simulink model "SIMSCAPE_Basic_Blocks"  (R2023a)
settings: Solver=VariableStepAuto  StartTime=0.0  StopTime=10.0  RelTol=1e-3
model workspace (MAT data in the model file):
  xx = 'A'
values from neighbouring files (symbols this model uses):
  R = 1    [Electrical_Transformer_EQN.m]    (also in Electrical_Transformer_SLX_m.m; Mechanical_Transmission_EQN.m; Mechanical_Transmission_SLX_m.m; Mechanical_system_EQN.m)
undefined symbols (not defined in the file or in its folder): Ap, eTr, mGi
libraries: fl_lib x28, nesl_utility x4

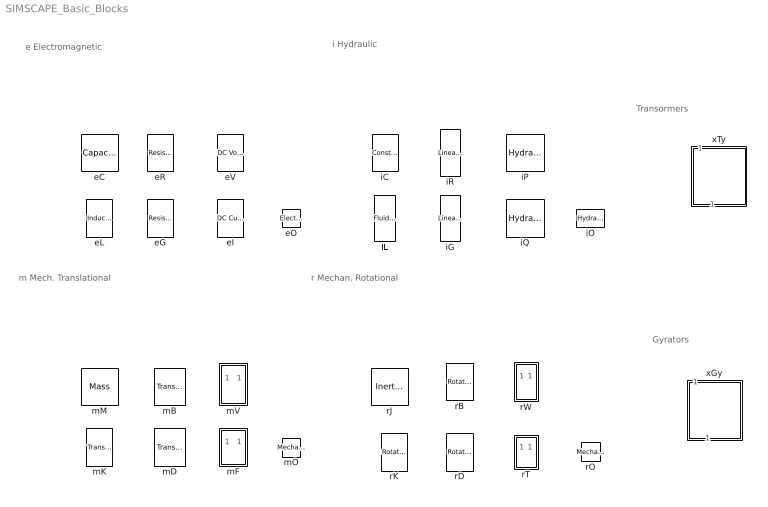
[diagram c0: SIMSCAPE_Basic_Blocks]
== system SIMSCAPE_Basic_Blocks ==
  note: m Mech. Translational
  note: r Mechan. Rotational
  note: i Hydraulic
  note: e Electromagnetic
  note: Transormers
  note: Gyrators
  eC : fl_lib/Electrical/Electrical Elements/Capacitor  c=1e-6 F  r=1e-6 Ohm  g=0 1/Ohm  i_specify=off  i_priority=None  i=0 A  i_nominal_specify=off  i_nominal_unit=A  i_nominal_value=1  v_specify=off  v_priority=None  v=0 V  v_nominal_specify=off  v_nominal_unit=V  v_nominal_value=1  vc_specify=off  vc_priority=High  vc=0 V  vc_nominal_specify=off  vc_nominal_unit=V  vc_nominal_value=1
  eG : fl_lib/Electrical/Electrical Elements/Resistor  R=1 Ohm  i_specify=off  i_priority=None  i=0 A  i_nominal_specify=off  i_nominal_unit=A  i_nominal_value=1  v_specify=off  v_priority=None  v=0 V  v_nominal_specify=off  v_nominal_unit=V  v_nominal_value=1
  eI : fl_lib/Electrical/Electrical Sources/DC Current Source  i0=1 A
  eL : fl_lib/Electrical/Electrical Elements/Inductor  l=1e-6 H  r=0 Ohm  g=1e-9 1/Ohm  i_specify=off  i_priority=None  i=0 A  i_nominal_specify=off  i_nominal_unit=A  i_nominal_value=1  v_specify=off  v_priority=None  v=0 V  v_nominal_specify=off  v_nominal_unit=V  v_nominal_value=1  i_L_specify=off  i_L_priority=High  i_L=0 A  i_L_nominal_specify=off  i_L_nominal_unit=A  i_L_nominal_value=1
  eO : fl_lib/Electrical/Electrical Elements/Electrical Reference
  eR : fl_lib/Electrical/Electrical Elements/Resistor  R=1 Ohm  i_specify=off  i_priority=None  i=0 A  i_nominal_specify=off  i_nominal_unit=A  i_nominal_value=1  v_specify=off  v_priority=None  v=0 V  v_nominal_specify=off  v_nominal_unit=V  v_nominal_value=1
  eV : fl_lib/Electrical/Electrical Sources/DC Voltage Source  v0=1 V
  iC : fl_lib/Hydraulic/Hydraulic Elements/Constant Volume Hydraulic Chamber  ch_sp=foundation.enum.chamberGeometry.volume  wall_type=foundation.enum.chamber_spec.rigid  ch_volume=1e-4 m^3  d_in=1e-2 m  length=1 m  pr_r_coef=1.2e-12 m/Pa  time_const=0.01 s  k_sh=1.4  pressure_specify=off  pressure_priority=High  pressure=0 Pa  pressure_nominal_specify=off  pressure_nominal_unit=Pa  pressure_nominal_value=1  diameter_incr_specify=off  diameter_incr_priority=High  diameter_incr=0 m  diameter_incr_nominal_specify=off  diameter_incr_nominal_unit=m  diameter_incr_nominal_value=1  flow_rate_specify=off  flow_rate_priority=None  flow_rate=1e-3 m^3/s  flow_rate_nominal_specify=off  flow_rate_nominal_unit=m^3/s  flow_rate_nominal_value=1
  iG : fl_lib/Hydraulic/Hydraulic Elements/Linear Hydraulic Resistance  resistance=10e9 Pa*s/m^3  q_specify=off  q_priority=None  q=1e-3 m^3/s  q_nominal_specify=off  q_nominal_unit=m^3/s  q_nominal_value=1  p_specify=off  p_priority=None  p=0 Pa  p_nominal_specify=off  p_nominal_unit=Pa  p_nominal_value=1
  iL : fl_lib/Hydraulic/Hydraulic Elements/Fluid Inertia  area=0.8e-4 m^2  length=1 m  q_specify=off  q_priority=High  q=1e-3 m^3/s  q_nominal_specify=off  q_nominal_unit=m^3/s  q_nominal_value=1  p_specify=off  p_priority=None  p=0 Pa  p_nominal_specify=off  p_nominal_unit=Pa  p_nominal_value=1
  iO : fl_lib/Hydraulic/Hydraulic Elements/Hydraulic Reference
  iP : fl_lib/Hydraulic/Hydraulic Sources/Hydraulic Constant Pressure Source  commanded_pressure=10e5 Pa
  iQ : fl_lib/Hydraulic/Hydraulic Sources/Hydraulic Constant Flow Rate Source  commanded_flow_rate=0.001 m^3/s
  iR : fl_lib/Hydraulic/Hydraulic Elements/Linear Hydraulic Resistance  resistance=10e9 Pa*s/m^3  q_specify=off  q_priority=None  q=1e-3 m^3/s  q_nominal_specify=off  q_nominal_unit=m^3/s  q_nominal_value=1  p_specify=off  p_priority=None  p=0 Pa  p_nominal_specify=off  p_nominal_unit=Pa  p_nominal_value=1
  mB : fl_lib/Mechanical/Translational Elements/Translational Damper  D=100 N*s/m  v_specify=off  v_priority=None  v=0 m/s  v_nominal_specify=off  v_nominal_unit=m/s  v_nominal_value=1  f_specify=off  f_priority=None  f=0 N  f_nominal_specify=off  f_nominal_unit=N  f_nominal_value=1
  mD : fl_lib/Mechanical/Translational Elements/Translational Damper  D=100 N*s/m  v_specify=off  v_priority=None  v=0 m/s  v_nominal_specify=off  v_nominal_unit=m/s  v_nominal_value=1  f_specify=off  f_priority=None  f=0 N  f_nominal_specify=off  f_nominal_unit=N  f_nominal_value=1
  mF : Subsystem  mask{mF='Fa'}
      mask prompts: mF "Output variable"
  mK : fl_lib/Mechanical/Translational Elements/Translational Spring  spr_rate=1000 N/m  v_specify=off  v_priority=None  v=0 m/s  v_nominal_specify=off  v_nominal_unit=m/s  v_nominal_value=1  f_specify=off  f_priority=None  f=0 N  f_nominal_specify=off  f_nominal_unit=N  f_nominal_value=1  x_specify=off  x_priority=High  x=0 m  x_nominal_specify=off  x_nominal_unit=m  x_nominal_value=1
  mM : fl_lib/Mechanical/Translational Elements/Mass  mass=1 kg  num_ports=foundation.enum.numPorts2.one  v_specify=off  v_priority=High  v=0 m/s  v_nominal_specify=off  v_nominal_unit=m/s  v_nominal_value=1  f_specify=off  f_priority=None  f=0 N  f_nominal_specify=off  f_nominal_unit=N  f_nominal_value=1
  mO : fl_lib/Mechanical/Translational Elements/Mechanical Translational Reference
  mV : Subsystem  mask{mV='Va'}
      mask prompts: mV "Output variable"
  rB : fl_lib/Mechanical/Rotational Elements/Rotational Damper  D=0.001 N*m*s/rad  w_specify=off  w_priority=None  w=0 rad/s  w_nominal_specify=off  w_nominal_unit=rad/s  w_nominal_value=1  t_specify=off  t_priority=None  t=0 N*m  t_nominal_specify=off  t_nominal_unit=N*m  t_nominal_value=1
  rD : fl_lib/Mechanical/Rotational Elements/Rotational Damper  D=0.001 N*m*s/rad  w_specify=off  w_priority=None  w=0 rad/s  w_nominal_specify=off  w_nominal_unit=rad/s  w_nominal_value=1  t_specify=off  t_priority=None  t=0 N*m  t_nominal_specify=off  t_nominal_unit=N*m  t_nominal_value=1
  rJ : fl_lib/Mechanical/Rotational Elements/Inertia  inertia=0.01 kg*m^2  num_ports=foundation.enum.numPorts2.one  w_specify=off  w_priority=High  w=0 rad/s  w_nominal_specify=off  w_nominal_unit=rad/s  w_nominal_value=1  t_specify=off  t_priority=None  t=0 N*m  t_nominal_specify=off  t_nominal_unit=N*m  t_nominal_value=1
  rK : fl_lib/Mechanical/Rotational Elements/Rotational Spring  spr_rate=10 N*m/rad  w_specify=off  w_priority=None  w=0 rad/s  w_nominal_specify=off  w_nominal_unit=rad/s  w_nominal_value=1  t_specify=off  t_priority=None  t=0 N*m  t_nominal_specify=off  t_nominal_unit=N*m  t_nominal_value=1  phi_specify=off  phi_priority=High  phi=0 rad  phi_nominal_specify=off  phi_nominal_unit=rad  phi_nominal_value=1
  rO : fl_lib/Mechanical/Rotational Elements/Mechanical Rotational Reference
  rT : Subsystem  mask{rT='Ta'}
      mask prompts: rT "Output variable"
  rW : Subsystem  mask{rW='Wa'}
      mask prompts: rW "Output variable"
  xGy : Subsystem  mask{Gyrator_type=mGi, G_type=F2=K*E1, xGy=Ap}
      mask prompts: Gyrator_type "Type of Gytator"; G_type "Type of relation"; xGy "Name of parameter K"
  xTy : Subsystem  mask{Transformer_type=eTr, T_type=E2=K*E1, xTy=R}
      mask prompts: Transformer_type "Type of Transformer"; T_type "Type of relation"; xTy "Name of parameter K"

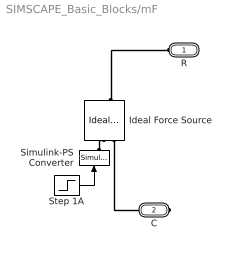
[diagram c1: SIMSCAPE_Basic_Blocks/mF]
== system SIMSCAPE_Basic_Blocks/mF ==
  Ideal Force Source : fl_lib/Mechanical/Mechanical Sources/Ideal Force Source
  Simulink-PS Converter : nesl_utility/Simulink-PS Converter  PhysicalDomain=network_engine_domain  SubClassName=ps_input  LeftPortType=input  RightPortType=output  PseudoPeriodic=off  Frequencies=[]  NoiseDistribution=none  NoiseParameters=[]  Unit=1  AffineConversion=off  FilteringAndDerivatives=zero  SimscapeFilterOrder=1  InputFilterTimeConstant=.001  UdotUserProvided=0
  Step 1A : Step  After=100  SampleTime=0
  R : PMIOPort  Side=Left
  C : PMIOPort  Port=2  Side=Right
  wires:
  Step 1A/1 -> Simulink-PS Converter/1
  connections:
  Ideal Force Source/RConn2 -- C/RConn1
  Ideal Force Source/LConn1 -- R/RConn1
  Simulink-PS Converter/RConn1 -- Ideal Force Source/RConn1

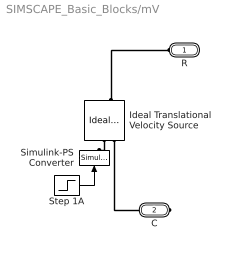
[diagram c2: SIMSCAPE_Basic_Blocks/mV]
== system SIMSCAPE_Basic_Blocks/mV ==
  Ideal Translational Velocity Source : fl_lib/Mechanical/Mechanical Sources/Ideal Translational Velocity Source
  Simulink-PS Converter : nesl_utility/Simulink-PS Converter  PhysicalDomain=network_engine_domain  SubClassName=ps_input  LeftPortType=input  RightPortType=output  PseudoPeriodic=off  Frequencies=[]  NoiseDistribution=none  NoiseParameters=[]  Unit=1  AffineConversion=off  FilteringAndDerivatives=zero  SimscapeFilterOrder=1  InputFilterTimeConstant=.001  UdotUserProvided=0
  Step 1A : Step  After=100  SampleTime=0
  R : PMIOPort  Side=Left
  C : PMIOPort  Port=2  Side=Right
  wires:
  Step 1A/1 -> Simulink-PS Converter/1
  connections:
  Ideal Translational Velocity Source/RConn2 -- C/RConn1
  Ideal Translational Velocity Source/LConn1 -- R/RConn1
  Ideal Translational Velocity Source/RConn1 -- Simulink-PS Converter/RConn1

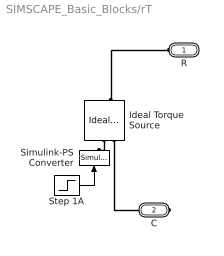
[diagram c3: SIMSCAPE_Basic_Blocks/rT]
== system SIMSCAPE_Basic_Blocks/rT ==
  Ideal Torque Source : fl_lib/Mechanical/Mechanical Sources/Ideal Torque Source
  Simulink-PS Converter : nesl_utility/Simulink-PS Converter  PhysicalDomain=network_engine_domain  SubClassName=ps_input  LeftPortType=input  RightPortType=output  PseudoPeriodic=off  Frequencies=[]  NoiseDistribution=none  NoiseParameters=[]  Unit=1  AffineConversion=off  FilteringAndDerivatives=zero  SimscapeFilterOrder=1  InputFilterTimeConstant=.001  UdotUserProvided=0
  Step 1A : Step  After=100  SampleTime=0
  R : PMIOPort  Side=Left
  C : PMIOPort  Port=2  Side=Right
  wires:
  Step 1A/1 -> Simulink-PS Converter/1
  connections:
  Ideal Torque Source/RConn1 -- Simulink-PS Converter/RConn1
  Ideal Torque Source/LConn1 -- R/RConn1
  Ideal Torque Source/RConn2 -- C/RConn1

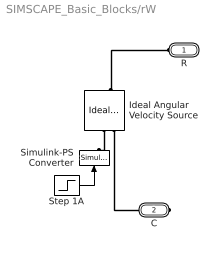
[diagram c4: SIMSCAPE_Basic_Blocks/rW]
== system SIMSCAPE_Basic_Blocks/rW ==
  Ideal Angular Velocity Source : fl_lib/Mechanical/Mechanical Sources/Ideal Angular Velocity Source
  Simulink-PS Converter : nesl_utility/Simulink-PS Converter  PhysicalDomain=network_engine_domain  SubClassName=ps_input  LeftPortType=input  RightPortType=output  PseudoPeriodic=off  Frequencies=[]  NoiseDistribution=none  NoiseParameters=[]  Unit=1  AffineConversion=off  FilteringAndDerivatives=zero  SimscapeFilterOrder=1  InputFilterTimeConstant=.001  UdotUserProvided=0
  Step 1A : Step  After=100  SampleTime=0
  R : PMIOPort  Side=Left
  C : PMIOPort  Port=2  Side=Right
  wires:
  Step 1A/1 -> Simulink-PS Converter/1
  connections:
  Ideal Angular Velocity Source/RConn2 -- C/RConn1
  Ideal Angular Velocity Source/LConn1 -- R/RConn1
  Ideal Angular Velocity Source/RConn1 -- Simulink-PS Converter/RConn1

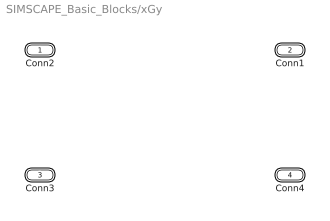
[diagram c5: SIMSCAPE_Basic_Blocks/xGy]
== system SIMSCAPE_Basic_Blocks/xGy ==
  Conn2 : PMIOPort  Side=Left
  Conn1 : PMIOPort  Port=2  Side=Left
  Conn3 : PMIOPort  Port=3  Side=Right
  Conn4 : PMIOPort  Port=4  Side=Right

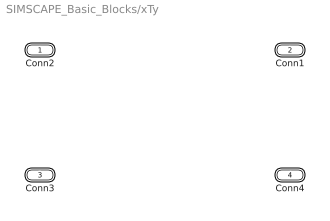
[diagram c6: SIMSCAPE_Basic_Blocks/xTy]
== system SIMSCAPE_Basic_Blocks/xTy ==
  Conn2 : PMIOPort  Side=Left
  Conn1 : PMIOPort  Port=2  Side=Left
  Conn3 : PMIOPort  Port=3  Side=Right
  Conn4 : PMIOPort  Port=4  Side=Right
